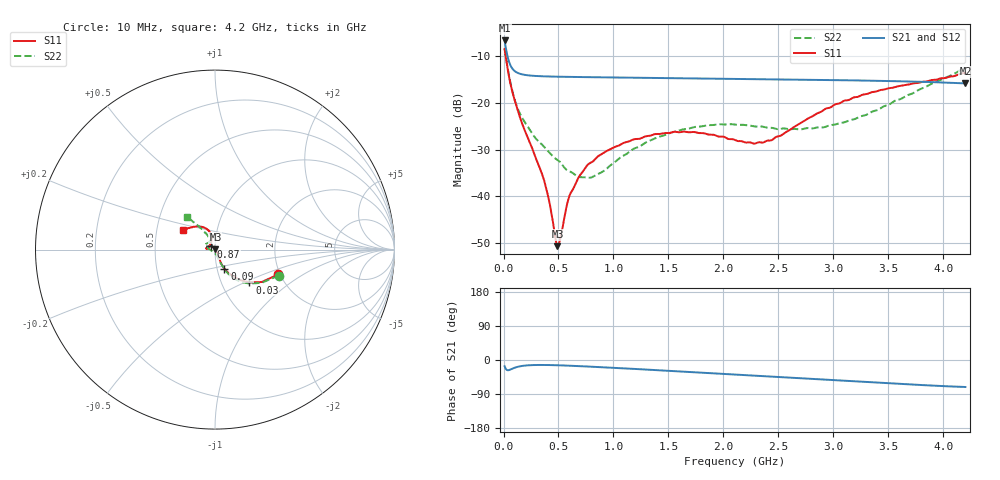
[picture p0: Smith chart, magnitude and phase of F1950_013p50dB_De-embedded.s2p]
! Integrated Device Technology
! Corporate Headquarters
! 6024 Silver Creek Valley Road
! San Jose, CA 95138  USA
! Phone:  1-408-284-8200
! Toll Free:  1-800-223-1366
! Webpage:  http://www.idt.com/
! Timing and RF Division
! 515 Groton Road, Suite 102
! Westford, MA 01886-6024
! Device:  F1950
! Description: 7-bit 0.25 dB Digital Step Attenuator
! Frequency:  150.0 -  4000.00 MHz
! Package:  4x4 mm Thin QFN Plastic Package: 24 pin
! Ports:  2 RF, 12 DC
!  Pin  1  = D0
!  Pin  2  = VDD
!  Pin  3  = Vmode
!  Pin  4  = GND
!  Pin  5  = RF1  =  Port 1
!  Pin  6  = GND
!  Pin  7  = GND
!  Pin  8  = GND
!  Pin  9  = GND
!  Pin 10  = GND
!  Pin 11  = GND
!  Pin 12  = GND
!  Pin 13  = GND
!  Pin 14  = RF2  =  Port 2
!  Pin 15  = GND
!  Pin 16  = LE
!  Pin 17  = CLK
!  Pin 18  = DATE
!  Pin 19  = D6
!  Pin 20  = D5
!  Pin 21  = D4
!  Pin 22  = D3
!  Pin 23  = D2
!  Pin 24  = D1
! State:  54
! Atten State:  13.50 dB
! Voltage:  +5.00 Volts
! Current:  Not Measured mA
! Data:  The device was measured on a the F195X evaluation board which has
!  individual transmission lines to the RF pins.  Data was collected
!  using a calibrated network analyzer.  The evaluation board was
!  de-embedded using a TRL calibration technique.
!  The reference plane is the edge of the package pin.
! Misc:  Board 2019
!  Action Tracker AT0250
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# GHz S dB R 50
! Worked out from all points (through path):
!   420 points, 10 MHz to 4.2 GHz, reference 50 ohm
!   highest |S21| = -6.59 dB at 10 MHz (marker M1); lowest = -15.8 dB at 4.2 GHz (marker M2)
!   group delay of S21, straight-line fit = 41.6 ps
!   lowest |S11| = -50.6 dB at 490 MHz (marker M3), VSWR 1.01, Z = 50.2 + j0.181 ohm
!   |S11| at or under -10 dB: 20.06 MHz to end of sweep
!   |S22| runs from -36.0 to -8.3 dB; largest |S21 - S12| = 0.00028
!   S11 on the Smith chart (normalised r, x): 10 MHz: 1.96, -0.63; 30 MHz: 1.35, -0.53; 90 MHz: 1.08, -0.24; 870 MHz: 0.96, +0.03; 4.2 GHz: 0.68, +0.16
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0.01  -8.41 -21.3  -6.59 -16.5  -6.59 -16.5  -8.33 -22.2
0.03  -11.53 -43.7  -9.26 -26.3  -9.26 -26.3  -11.43 -45.0
0.05  -14.34 -54.5  -11.13 -26.6  -11.13 -26.6  -14.12 -56.0
0.09  -18.45 -63.8  -12.89 -21.7  -12.89 -21.7  -18.34 -63.8
0.18  -25.07 -64.1  -13.90 -15.2  -13.90 -15.3  -23.58 -69.7
0.37  -36.61 -47.7  -14.28 -13.1  -14.28 -13.1  -29.38 -74.5
0.42  -41.52 -39.2  -14.31 -13.3  -14.31 -13.4  -30.67 -75.9
0.47  -48.69 -0.0  -14.34 -13.7  -14.34 -13.7  -31.84 -81.8
0.49  -50.65 37.8  -14.35 -13.9  -14.35 -13.9  -32.17 -83.5
0.52  -48.55 84.4  -14.36 -14.1  -14.36 -14.2  -32.77 -84.7
0.6  -39.83 118.6  -14.39 -15.0  -14.39 -15.0  -34.65 -97.3
0.71  -35.02 129.8  -14.43 -16.4  -14.43 -16.4  -35.86 -116.9
0.87  -31.23 140.7  -14.48 -18.7  -14.48 -18.7  -35.07 -150.6
1.1  -28.46 153.3  -14.55 -22.1  -14.55 -22.1  -31.14 -178.6
1.41  -26.62 166.6  -14.63 -27.0  -14.63 -27.0  -27.24 167.0
1.73  -26.19 173.8  -14.71 -32.2  -14.71 -32.2  -25.17 158.1
2.11  -27.98 164.8  -14.81 -38.5  -14.81 -38.5  -24.63 148.5
2.43  -28.00 129.8  -14.89 -43.7  -14.89 -43.7  -25.29 138.3
2.81  -22.82 106.0  -15.00 -50.2  -15.00 -50.2  -25.43 122.5
3.11  -19.43 108.5  -15.11 -55.2  -15.10 -55.3  -24.04 117.0
3.51  -16.80 119.1  -15.28 -61.7  -15.28 -61.7  -20.27 118.6
4.2  -13.48 148.4  -15.79 -71.3  -15.78 -71.3  -12.43 130.4
